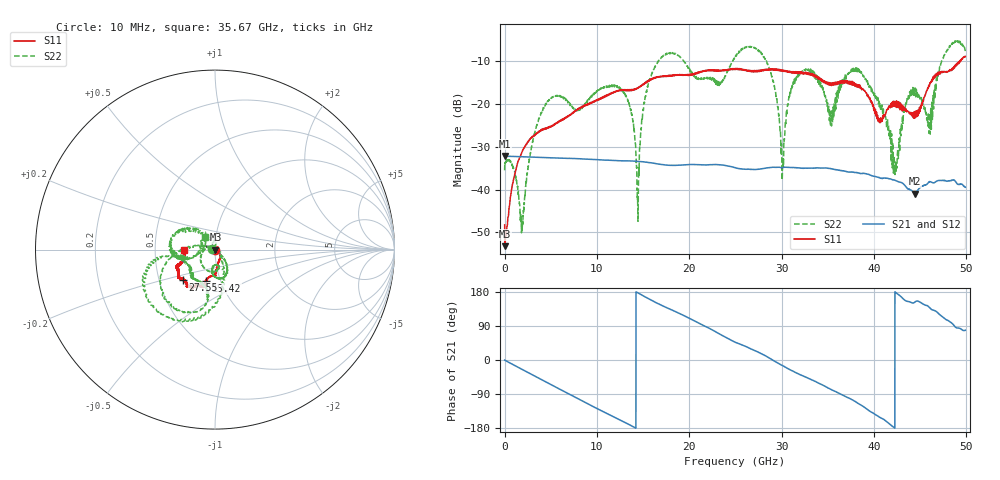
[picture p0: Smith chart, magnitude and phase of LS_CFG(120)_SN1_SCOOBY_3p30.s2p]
!Keysight Technologies,N5245B,MY58422026,A.13.80.08
!Date: Friday, March 20, 2020 00:04:53
!Correction: S11(Full 2 Port(1,2))
!S21(Full 2 Port(1,2))
!S12(Full 2 Port(1,2))
!S22(Full 2 Port(1,2))
!S2P File: Measurements: S11, S21, S12, S22:
# Hz S DB R 50.0
!freq dBS11 angS11 dBS21 angS21 dBS12 angS12 dBS22 angS22
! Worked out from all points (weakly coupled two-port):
!   4991 points, 10 MHz to 49.91 GHz, reference 50 ohm
!   highest |S21| = -32.13 dB at 20 MHz (marker M1); lowest = -40.9 dB at 44.42 GHz (marker M2)
!   lowest |S11| = -53.2 dB at 30 MHz (marker M3), VSWR 1.00, Z = 50.2 - j0.0279 ohm
!   |S11| at or under -10 dB: start of sweep to 49.25 GHz; 49.28459 GHz to 49.34289 GHz (58.29 MHz wide, 0.118 % of centre)
!   |S22| runs from -50.1 to -5.1 dB; largest |S21 - S12| = 0.00027
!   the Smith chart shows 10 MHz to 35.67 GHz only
!   S11 on the Smith chart (normalised r, x): 10 MHz: 1.01, -0.01; 15.42 GHz: 0.86, -0.31; 27.55 GHz: 0.66, -0.24; 35.67 GHz: 0.71, -0.00
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1e7  -48.26 -48.4  -32.15 -0.2  -32.15 -0.3  -35.49 177.0
2e7  -52.58 -23.3  -32.13 -0.4  -32.15 -0.5  -34.13 -178.9
3e7  -53.23 -7.3  -32.16 -0.5  -32.16 -0.5  -33.94 -176.2
1.91e9  -31.14 -40.2  -32.30 -24.9  -32.28 -24.9  -49.51 9.1
4.27e9  -25.78 -53.9  -32.50 -55.2  -32.49 -55.1  -20.73 -150.2
8.33e9  -20.83 -80.3  -32.80 -107.2  -32.81 -107.1  -20.96 -93.3
1.276e10  -16.77 -88.8  -33.26 -161.3  -33.25 -161.2  -16.80 -63.3
1.444e10  -16.24 -100.5  -33.38 177.2  -33.37 177.3  -46.56 -96.0
1.542e10  -14.89 -105.7  -33.60 164.2  -33.60 164.3  -16.67 174.2
1.665e10  -13.68 -105.7  -34.01 148.5  -34.00 148.6  -9.99 -157.4
2.496e10  -11.83 -127.7  -34.84 47.2  -34.83 47.5  -9.09 -167.8
2.755e10  -12.19 -136.6  -35.21 19.8  -35.21 20.1  -7.62 -110.2
3.011e10  -12.31 -145.4  -34.83 -14.6  -34.84 -14.3  -34.79 14.3
3.116e10  -12.49 -149.7  -34.84 -28.5  -34.86 -28.1  -15.61 140.4
3.328e10  -13.05 -158.6  -34.96 -52.6  -34.98 -52.2  -12.32 -175.2
3.567e10  -15.38 -179.7  -35.25 -81.3  -35.20 -80.9  -20.88 128.1
3.816e10  -15.96 175.9  -36.04 -112.5  -35.98 -112.6  -11.56 -174.7
4.16e10  -20.59 102.8  -37.43 -166.9  -37.46 -166.9  -25.60 67.5
4.233e10  -19.64 103.8  -37.86 179.0  -37.88 179.0  -33.75 164.0
4.442e10  -23.31 51.7  -40.94 152.4  -40.97 152.7  -17.80 -10.9
4.601e10  -15.78 2.9  -38.13 138.4  -38.15 138.7  -23.26 116.8
4.991e10  -8.85 -13.7  -39.43 78.5  -39.45 78.6  -7.37 -14.7
